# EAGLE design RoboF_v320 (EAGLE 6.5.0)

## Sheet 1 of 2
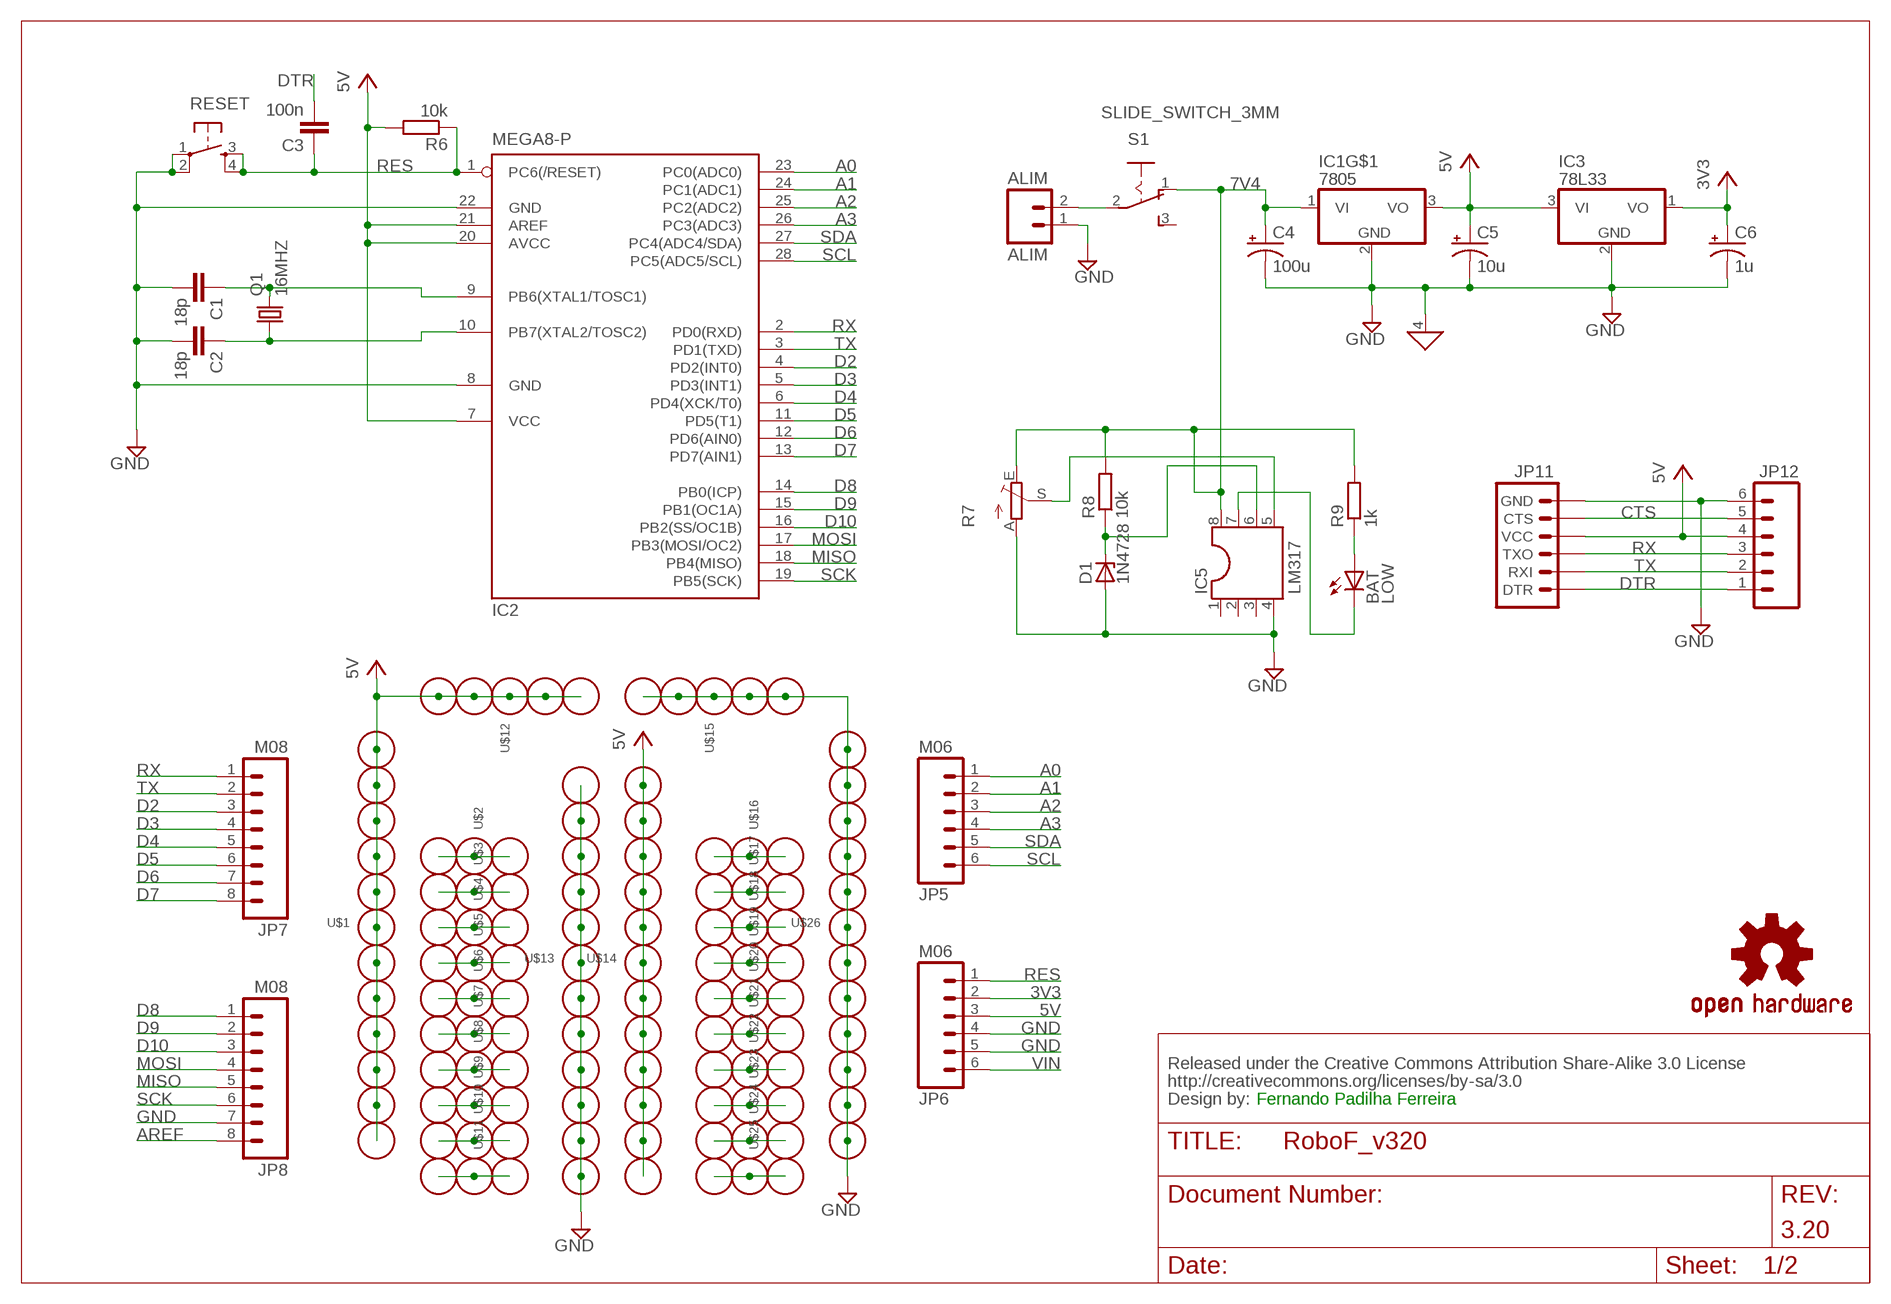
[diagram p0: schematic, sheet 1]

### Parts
ALIM  ALIM  M02POLAR  [MOLEX-1X2]
BAT  LOW  TLLG4400  [LED3MM]
C1  18p  C-EU050-024X044  [C050-024X044]
C2  18p  C-EU050-024X044  [C050-024X044]
C3  100n  C-EU050-024X044  [C050-024X044]
C4  100u  CPOL-USE2.5-6  [E2,5-6]
C5  10u  CPOL-USE2.5-6  [E2,5-6]
C6  1u  CPOL-USE2.5-5  [E2,5-5]
CC_TEXT1  CREATIVE_COMMONS  [CREATIVE_COMMONS]
D1  1N4728  [DO41Z10]
IC1  7805  [TO220H]
IC2  MEGA8-P  [DIL28-3]
IC3  78L33  78L24Z  [TO92]
IC5  LM317  DIL8  [DIL08]
JP5  M06  [1X06_FEMALE_NO_SILK]
JP6  M06  [1X06_FEMALE_NO_SILK]
JP7  M08  [1X08_FEMALE_NO_SILK]
JP8  M08  [1X08_FEMALE_NO_SILK]
JP11  ARDUINO_SERIAL_PROGRAMPTH  [1X06]
JP12  M06SIP  [1X06]
LOGO1  OSHW-LOGOL  [OSHW-LOGO-L]
Q1  16MHZ  CRYSTALHC49S  [HC49/S]
R6  10k  R-EU_0207/7  [0207/7]
R7  TRIM_EU-RS3  [RS3]
R8  10k  R-EU_0207/7  [0207/7]
R9  1k  R-EU_0207/7  [0207/7]
RESET  TAC_SWITCHPTH  [TACTILE-PTH]
S1  SLIDE_SWITCH_3MM  [SS3MM]
U$1  WIREPAD-12X1  [12X-1,6/0,9]
U$2  WIREPAD-3X1  [3X-1,6/0,9]
U$3  WIREPAD-3X1  [3X-1,6/0,9]
U$4  WIREPAD-3X1  [3X-1,6/0,9]
U$5  WIREPAD-3X1  [3X-1,6/0,9]
U$6  WIREPAD-3X1  [3X-1,6/0,9]
U$7  WIREPAD-3X1  [3X-1,6/0,9]
U$8  WIREPAD-3X1  [3X-1,6/0,9]
U$9  WIREPAD-3X1  [3X-1,6/0,9]
U$10  WIREPAD-3X1  [3X-1,6/0,9]
U$11  WIREPAD-3X1  [3X-1,6/0,9]
U$12  WIREPAD-5X1  [5X-1,6/0,9]
U$13  WIREPAD-12X1  [12X-1,6/0,9]
U$14  WIREPAD-12X1  [12X-1,6/0,9]
U$15  WIREPAD-5X1  [5X-1,6/0,9]
U$16  WIREPAD-3X1  [3X-1,6/0,9]
U$17  WIREPAD-3X1  [3X-1,6/0,9]
U$18  WIREPAD-3X1  [3X-1,6/0,9]
U$19  WIREPAD-3X1  [3X-1,6/0,9]
U$20  WIREPAD-3X1  [3X-1,6/0,9]
U$21  WIREPAD-3X1  [3X-1,6/0,9]
U$22  WIREPAD-3X1  [3X-1,6/0,9]
U$23  WIREPAD-3X1  [3X-1,6/0,9]
U$24  WIREPAD-3X1  [3X-1,6/0,9]
U$25  WIREPAD-3X1  [3X-1,6/0,9]
U$26  WIREPAD-12X1  [12X-1,6/0,9]

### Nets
3V3: C6.+ IC3.1(VO) JP6.2 ; also sheet 2
5V: C5.+ IC1.3(VO) IC2.7(VCC) IC2.20(AVCC) IC2.21(AREF) IC3.3(VI) JP6.3 JP11.4(VCC) JP12.4 R6.2 U$1.P$1 U$1.P$2 U$1.P$3 U$1.P$4 U$1.P$5 U$1.P$6 U$1.P$7 U$1.P$8 U$1.P$9 U$1.P$10 U$1.P$11 U$1.P$12 U$12.P$1(P$) U$12.P$2 U$12.P$3 U$12.P$4 U$12.P$5 U$14.P$1 U$14.P$2 U$14.P$3 U$14.P$4 U$14.P$5 U$14.P$6 U$14.P$7 U$14.P$8 U$14.P$9 U$14.P$10 U$14.P$11 U$14.P$12 ; also sheet 2
7V4 [MTR]: C4.+ IC1.1(VI) IC5.8 R7.E R8.2 R9.2 S1.1(O) ; also sheet 2
A0 [SIGNAL]: IC2.23(PC0(ADC0)) JP5.1 ; also sheet 2
A1 [SIGNAL]: IC2.24(PC1(ADC1)) JP5.2 ; also sheet 2
A2 [SIGNAL]: IC2.25(PC2(ADC2)) JP5.3 ; also sheet 2
A3 [SIGNAL]: IC2.26(PC3(ADC3)) JP5.4 ; also sheet 2
AREF: JP8.8
CTS [SIGNAL]: JP11.5(CTS) JP12.5
D2 [SIGNAL]: IC2.4(PD2(INT0)) JP7.3 ; also sheet 2
D3 [SIGNAL]: IC2.5(PD3(INT1)) JP7.4 ; also sheet 2
D4 [SIGNAL]: IC2.6(PD4(XCK/T0)) JP7.5 ; also sheet 2
D5 [SIGNAL]: IC2.11(PD5(T1)) JP7.6 ; also sheet 2
D6 [SIGNAL]: IC2.12(PD6(AIN0)) JP7.7 ; also sheet 2
D7 [SIGNAL]: IC2.13(PD7(AIN1)) JP7.8 ; also sheet 2
D8 [SIGNAL]: IC2.14(PB0(ICP)) JP8.1 ; also sheet 2
D9 [SIGNAL]: IC2.15(PB1(OC1A)) JP8.2 ; also sheet 2
D10 [SIGNAL]: IC2.16(PB2(SS/OC1B)) JP8.3 ; also sheet 2
DTR [SIGNAL]: C3.2 JP11.1(DTR) JP12.1
GND: ALIM.1 C1.2 C2.2 C4.- C5.- C6.- D1.A IC1.2(GND) IC1.4(GND) IC2.8(GND) IC2.22(GND) IC3.2(GND) IC5.4 JP6.4 JP6.5 JP8.7 JP11.6(GND) JP12.6 R7.A RESET.1 RESET.2 U$13.P$1 U$13.P$2 U$13.P$3 U$13.P$4 U$13.P$5 U$13.P$6 U$13.P$7 U$13.P$8 U$13.P$9 U$13.P$10 U$13.P$11 U$13.P$12 U$15.P$1(P$) U$15.P$2 U$15.P$3 U$15.P$4 U$15.P$5 U$26.P$1 U$26.P$2 U$26.P$3 U$26.P$4 U$26.P$5 U$26.P$6 U$26.P$7 U$26.P$8 U$26.P$9 U$26.P$10 U$26.P$11 U$26.P$12 ; also sheet 2
GND1: BAT.K(C) IC5.7
MISO [SIGNAL]: IC2.18(PB4(MISO)) JP8.5 ; also sheet 2
MOSI [SIGNAL]: IC2.17(PB3(MOSI/OC2)) JP8.4 ; also sheet 2
N$6 [SIGNAL]: C2.1 IC2.10(PB7(XTAL2/TOSC2)) Q1.1
N$8 [MTR]: ALIM.2 S1.2(P)
N$11 [SIGNAL]: C1.1 IC2.9(PB6(XTAL1/TOSC1)) Q1.2
N$55: U$3.P$1 U$3.P$2 U$3.P$3
N$56: U$4.P$1 U$4.P$2 U$4.P$3
N$57: U$5.P$1 U$5.P$2 U$5.P$3
N$58: U$6.P$1 U$6.P$2 U$6.P$3
N$59: U$7.P$1 U$7.P$2 U$7.P$3
N$70: U$8.P$1 U$8.P$2 U$8.P$3
N$80: U$9.P$1 U$9.P$2 U$9.P$3
N$88: U$10.P$1 U$10.P$2 U$10.P$3
N$89: U$11.P$1 U$11.P$2 U$11.P$3
N$92: U$17.P$1 U$17.P$2 U$17.P$3
N$93: U$18.P$1 U$18.P$2 U$18.P$3
N$94: U$19.P$1 U$19.P$2 U$19.P$3
N$115: U$20.P$1 U$20.P$2 U$20.P$3
N$116: U$21.P$1 U$21.P$2 U$21.P$3
N$117: U$22.P$1 U$22.P$2 U$22.P$3
N$120: U$23.P$1 U$23.P$2 U$23.P$3
N$121: U$24.P$1 U$24.P$2 U$24.P$3
N$122: U$25.P$1 U$25.P$2 U$25.P$3
N$124: U$2.P$1 U$2.P$2 U$2.P$3
N$126: U$16.P$1 U$16.P$2 U$16.P$3
N$185 [SIGNAL]: BAT.A R9.1
N$189: D1.C IC5.6 R8.1
N$190: IC5.5 R7.S
RES [SIGNAL]: C3.1 IC2.1(PC6(/RESET)) JP6.1 R6.1 RESET.3 RESET.4 ; also sheet 2
RX [SIGNAL]: IC2.2(PD0(RXD)) JP7.1 JP11.3(TXO) JP12.3 ; also sheet 2
SCK [SIGNAL]: IC2.19(PB5(SCK)) JP8.6 ; also sheet 2
SCL [SIGNAL]: IC2.28(PC5(ADC5/SCL)) JP5.6 ; also sheet 2
SDA [SIGNAL]: IC2.27(PC4(ADC4/SDA)) JP5.5 ; also sheet 2
TX [SIGNAL]: IC2.3(PD1(TXD)) JP7.2 JP11.2(RXI) JP12.2 ; also sheet 2
VIN: JP6.6
Unconnected: IC5.1 IC5.2 IC5.3 S1.3(S)

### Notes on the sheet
- Fernando Padilha Ferreira
- 3.20

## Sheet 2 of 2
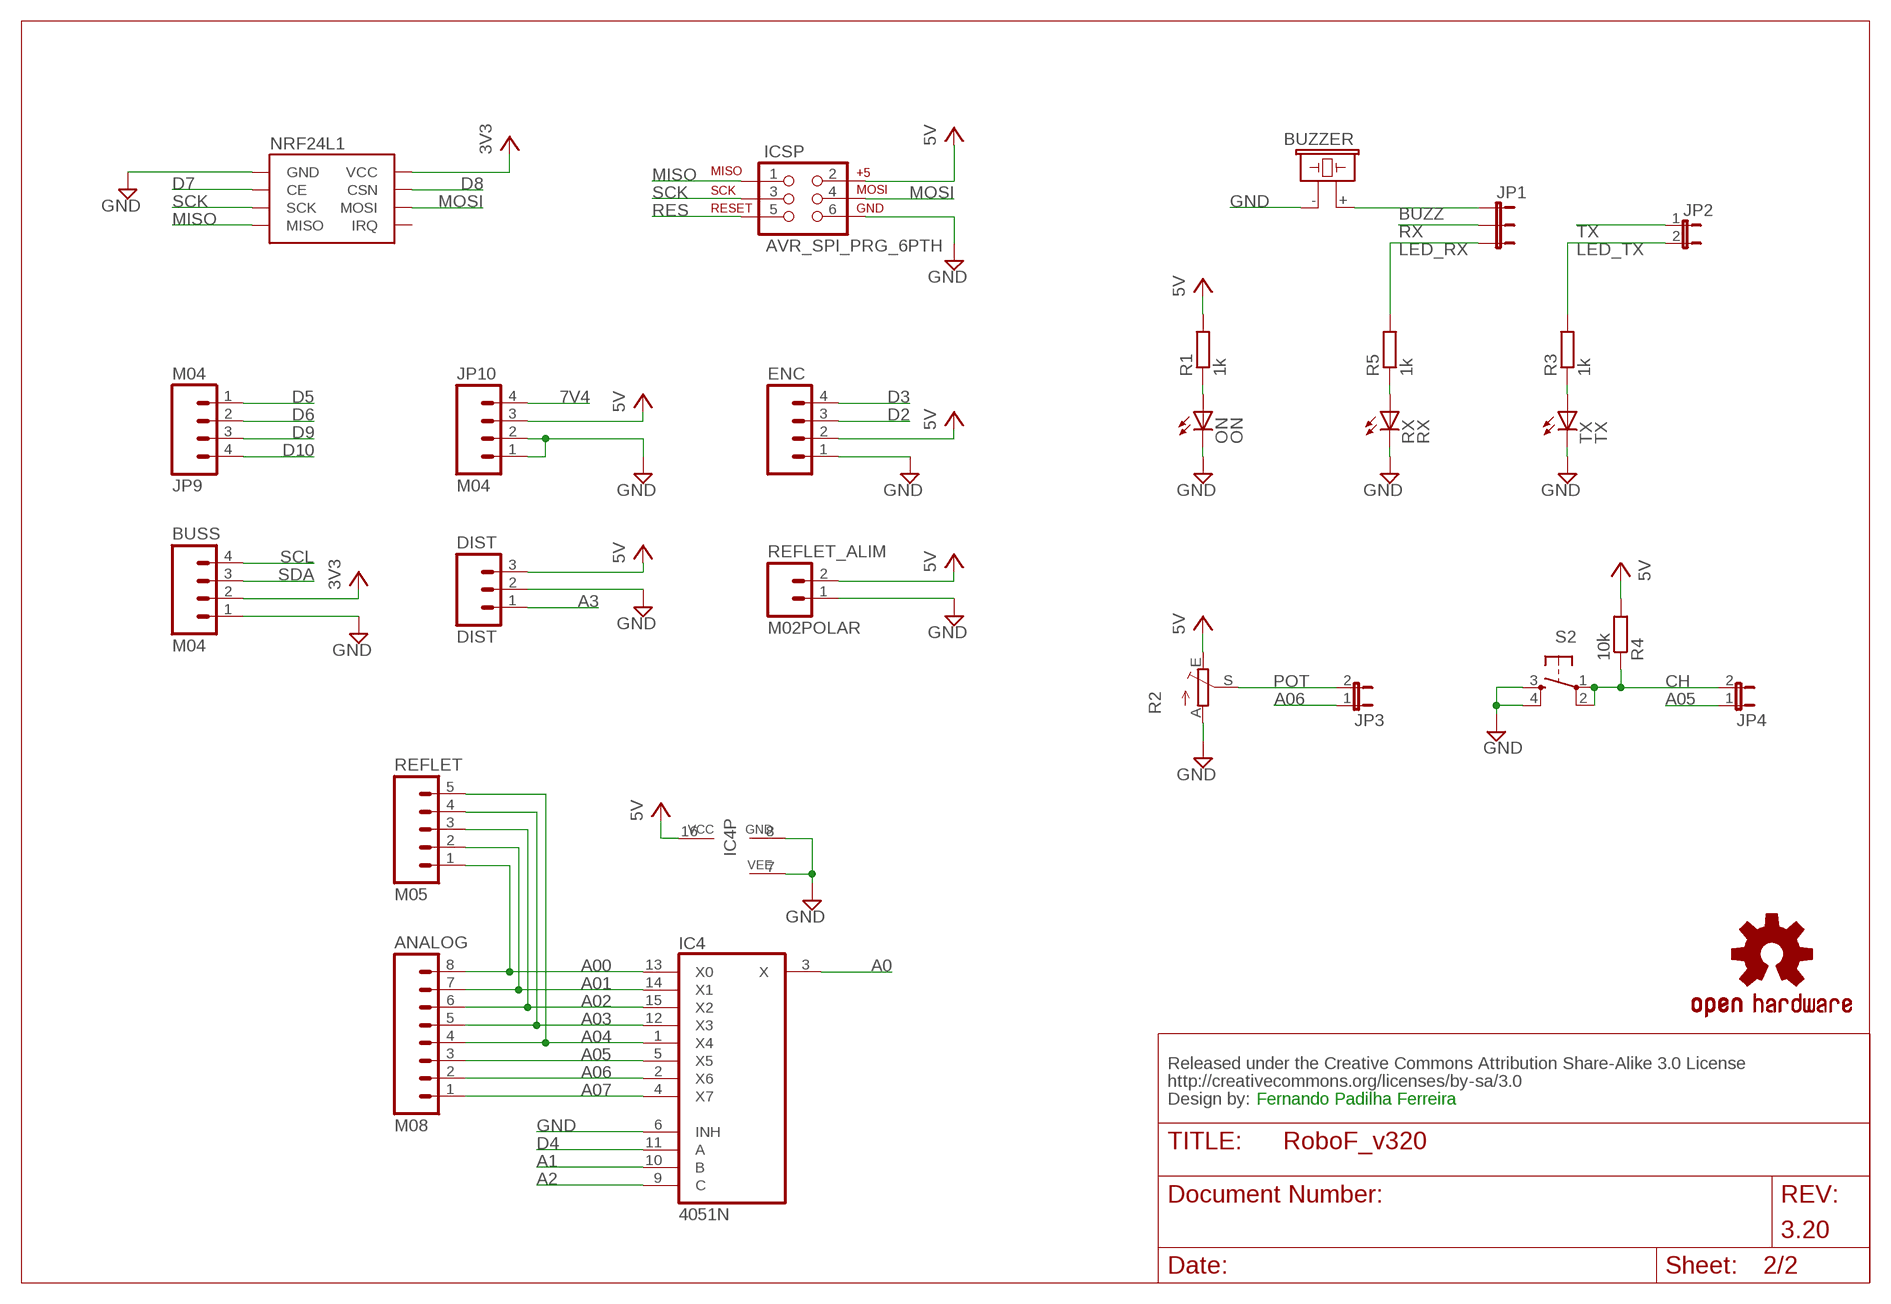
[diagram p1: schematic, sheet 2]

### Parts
ANALOG  M08  [1X08_FEMALE_NO_SILK]
BUSS  M04  [1X04_FEMALE]
BUZZER  F/CM12P  [F/CM12P]
CC_TEXT2  CREATIVE_COMMONS  [CREATIVE_COMMONS]
DIST  DIST  M03POLAR  [MOLEX-1X3]
ENC  M04POLAR  [MOLEX-1X4]
IC4  4051N  [DIL16]
ICSP  AVR_SPI_PRG_6PTH  [2X3]
JP1  JUMPER-3PTH  [1X03]
JP2  JUMPER-2PTH  [1X02]
JP3  JUMPER-2PTH  [1X02]
JP4  JUMPER-2PTH  [1X02]
JP9  M04  [1X04_FEMALE]
JP10  M04  [1X04_FEMALE]
LOGO2  OSHW-LOGOL  [OSHW-LOGO-L]
NRF24L1  NRF24L01  [NRF24L01]
ON  ON  TLLG4400  [LED3MM]
R1  1k  R-EU_0207/7  [0207/7]
R2  TRIM_EU-RS3  [RS3]
R3  1k  R-EU_0207/7  [0207/7]
R4  10k  R-EU_0207/7  [0207/7]
R5  1k  R-EU_0207/7  [0207/7]
REFLET  M05  [MOLEX-1X5]
REFLET_ALIM  M02POLAR  [MOLEX-1X2]
RX  RX  TLLR4400  [LED3MM]
S2  TAC_SWITCHPTH  [TACTILE-PTH]
TX  TX  TLLR4400  [LED3MM]

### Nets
3V3: BUSS.2 NRF24L1.2(VCC) ; also sheet 1
5V: DIST.3 ENC.2 IC4.16(VCC) ICSP.2 JP10.3 R1.2 R2.E R4.2 REFLET_ALIM.2 ; also sheet 1
7V4 [MTR]: JP10.4 ; also sheet 1
A0 [SIGNAL]: IC4.3(X) ; also sheet 1
A00 [SIGNAL]: ANALOG.8 IC4.13(X0) REFLET.1
A1 [SIGNAL]: IC4.10(B) ; also sheet 1
A01 [SIGNAL]: ANALOG.7 IC4.14(X1) REFLET.2
A2 [SIGNAL]: IC4.9(C) ; also sheet 1
A02 [SIGNAL]: ANALOG.6 IC4.15(X2) REFLET.3
A3 [SIGNAL]: DIST.1 ; also sheet 1
A03 [SIGNAL]: ANALOG.5 IC4.12(X3) REFLET.4
A04 [SIGNAL]: ANALOG.4 IC4.1(X4) REFLET.5
A05 [SIGNAL]: ANALOG.3 IC4.5(X5) JP4.1
A06 [SIGNAL]: ANALOG.2 IC4.2(X6) JP3.1
A07 [SIGNAL]: ANALOG.1 IC4.4(X7)
BUZZ [SIGNAL]: BUZZER.+ JP1.1
CH [SIGNAL]: JP4.2 R4.1 S2.1 S2.2
D2 [SIGNAL]: ENC.3 ; also sheet 1
D3 [SIGNAL]: ENC.4 ; also sheet 1
D4 [SIGNAL]: IC4.11(A) ; also sheet 1
D5 [SIGNAL]: JP9.1 ; also sheet 1
D6 [SIGNAL]: JP9.2 ; also sheet 1
D7 [SIGNAL]: NRF24L1.3(CE) ; also sheet 1
D8 [SIGNAL]: NRF24L1.4(CSN) ; also sheet 1
D9 [SIGNAL]: JP9.3 ; also sheet 1
D10 [SIGNAL]: JP9.4 ; also sheet 1
GND: BUSS.1 BUZZER.- DIST.2 ENC.1 IC4.6(INH) IC4.7(VEE) IC4.8(GND) ICSP.6 JP10.1 JP10.2 NRF24L1.1(GND) ON.K(C) R2.A REFLET_ALIM.1 RX.K(C) S2.3 S2.4 TX.K(C) ; also sheet 1
LED_RX [SIGNAL]: JP1.3 R5.2
LED_TX [SIGNAL]: JP2.2 R3.2
MISO [SIGNAL]: ICSP.1 NRF24L1.7(MISO) ; also sheet 1
MOSI [SIGNAL]: ICSP.4 NRF24L1.6(MOSI) ; also sheet 1
N$1 [SIGNAL]: R3.1 TX.A
N$2 [SIGNAL]: R5.1 RX.A
N$186 [SIGNAL]: ON.A R1.1
POT [SIGNAL]: JP3.2 R2.S
RES [SIGNAL]: ICSP.5 ; also sheet 1
RX [SIGNAL]: JP1.2 ; also sheet 1
SCK [SIGNAL]: ICSP.3 NRF24L1.5(SCK) ; also sheet 1
SCL [SIGNAL]: BUSS.4 ; also sheet 1
SDA [SIGNAL]: BUSS.3 ; also sheet 1
TX [SIGNAL]: JP2.1 ; also sheet 1
Unconnected: NRF24L1.8(IRQ)

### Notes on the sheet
- Fernando Padilha Ferreira
- 3.20

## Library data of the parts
ALIM = SparkFun:M02: Header 2
ANALOG JP7 JP8 = FernandoLib:M08
BAT ON = led:TLLG4400: Low Current (2mA) LED 3 mm Tinted Diffused Package color GREEN; MF: VISHAY SEMICONDUCTOR; OC_FARNELL: 1612435
BUSS JP9 JP10 = FernandoLib:M04
BUZZER = buzzer:F/CM12P: BUZZER; OC_FARNELL: unknown; OC_NEWARK: unknown
C1-C3 = rcl:C-EU: CAPACITOR, European symbol
C4 C5 = rcl:CPOL-US: POLARIZED CAPACITOR, American symbol
C6 = resistor:CPOL-US: POLARIZED CAPACITOR, American symbol
CC_TEXT1 CC_TEXT2 = SparkFun-Aesthetics:CREATIVE_COMMONS: Creative Commons License summary
D1 = diode:1N4728: Z DIODE
DIST = SparkFun-Connectors:M03: Header 3 Standard 3-pin 0.1" header. Use with straight break away headers (SKU : PRT-00116), right angle break away headers (PRT-00553), swiss pins (PRT-00743), machine pins (PRT-00117), and female headers (PRT-00115). Molex polarized connector foot print use with SKU : PRT-08232 with associated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
ENC = SparkFun-Connectors:M04: Header 4 Standard 4-pin 0.1" header. Use with straight break away headers (SKU : PRT-00116), right angle break away headers (PRT-00553), swiss pins (PRT-00743), machine pins (PRT-00117), and female headers (PRT-00115). Molex polarized connector foot print use with SKU : PRT-08231 with associated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
IC1 = FernandoLib:78*
IC2 = atmel:MEGA8-P: MICROCONTROLLER 8 Kbytes FLASH, 1 kbytes SRAM, 512 bytes EEPROM, USART, 4-channel 10 bit ADC, 2-channel 8 bit ADC Pin compatible with Atmega48, ATMega88, ATMega168 Source: avr.lbr; OC_FARNELL: unknown; OC_NEWARK: unknown
IC3 = linear:78*: Positive VOLTAGE REGULATOR Source: http://cache.national.com/ds/LM/LM78L05.pdf http://www.fairchildsemi.com/ds/LM/LM7805.pdf
IC4 = 40xx:4051: 8-channel ANALOG MULTIPLEXER
IC5 = ic-package:DIL8: Dual In Line / Socket
ICSP = SparkFun-Connectors:AVR_SPI_PRG_6: AVR ISP 6 Pin This is the reduced ISP connector for AVR programming. Common on Arduino. This footprint will take up less PCB space and can be used with a 10-pin to 6-pin adapter such as SKU: BOB-08508
JP1 = SparkFun-Passives:JUMPER-3
JP2-JP4 = SparkFun-Passives:JUMPER-2: Jumper
JP5 JP6 = FernandoLib:M06
JP11 = SparkFun-Connectors:ARDUINO_SERIAL_PROGRAM: FTDI connector footprints
JP12 = SparkFun-Connectors:M06: Header 6 Standard 6-pin 0.1" header. Use with straight break away headers (SKU : PRT-00116), right angle break away headers (PRT-00553), swiss pins (PRT-00743), machine pins (PRT-00117), and female headers (PRT-00115). Molex polarized connector foot print use with SKU : PRT-08094 with associated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
LOGO1 LOGO2 = SparkFun-Aesthetics:OSHW-LOGO: Open Source Hardware Logo This logo indicates the piece of hardware it is found on incorporates a OSHW license and/or adheres to the definition of open source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
NRF24L1 = FernandoLib:NRF24L01
Q1 = crystal:CRYSTAL: CRYSTAL; OC_FARNELL: 1667008; OC_NEWARK: unknown
R1 R3-R6 R8 R9 = resistor:R-EU_: RESISTOR, European symbol
R2 R7 = pot:TRIM_EU-: POTENTIOMETER
REFLET = FernandoLib:M05
REFLET_ALIM = SparkFun-Connectors:M02: Standard 2-pin 0.1" header. Use with
RESET S2 = SparkFun:TAC_SWITCH: Momentary Switch Button commonly used for reset or general input. Spark Fun Electronics SKU : COM-00097
RX TX = led:TLLR4400: Low Current (2mA) LED 3 mm Tinted Diffused Package color RED; MF: VISHAY SEMICONDUCTOR; OC_FARNELL: 1612437
S1 = FernandoLib:SLIDE_SWITCH_3MM
U$1 U$13 U$14 U$26 = FernandoLib:WIREPAD-12X1
U$2-U$11 U$16-U$25 = FernandoLib:WIREPAD-3X1
U$12 U$15 = FernandoLib:WIREPAD-5X1

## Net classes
0 GND: width 0.762 mm, clearance 0.406 mm
1 MTR: width 1.016 mm, clearance 0.406 mm

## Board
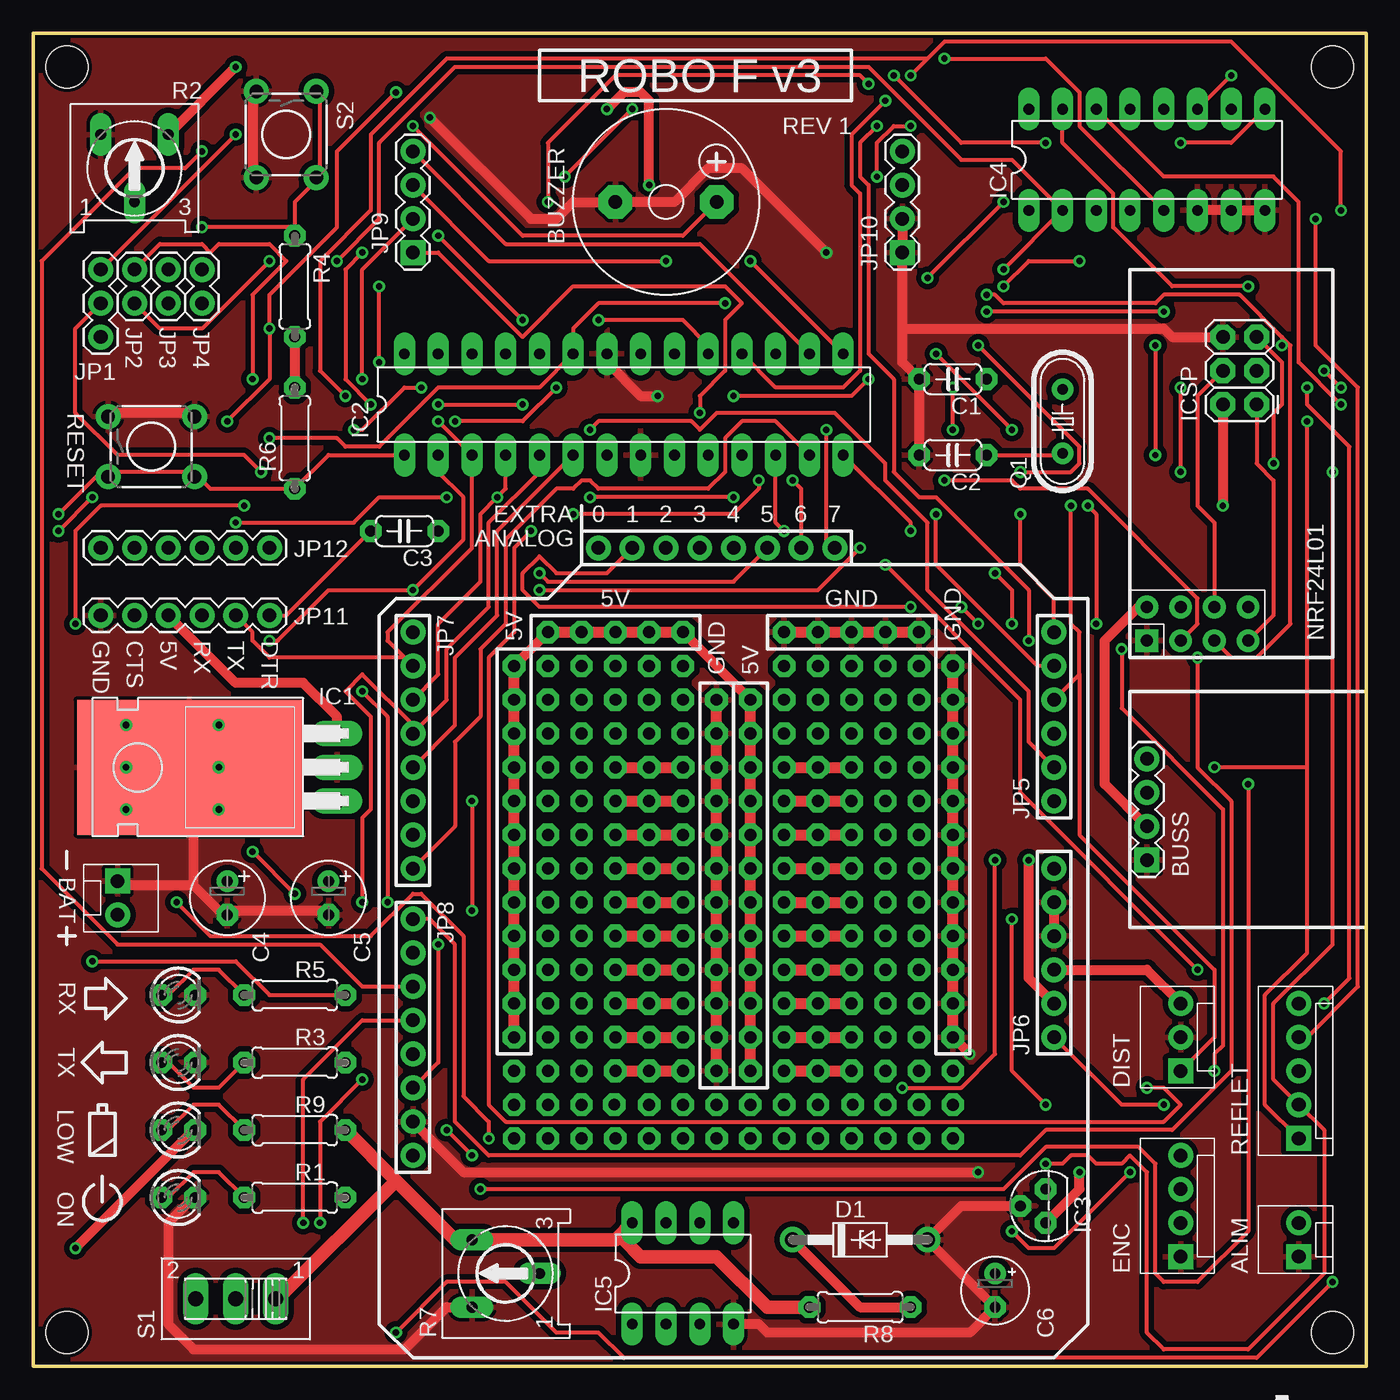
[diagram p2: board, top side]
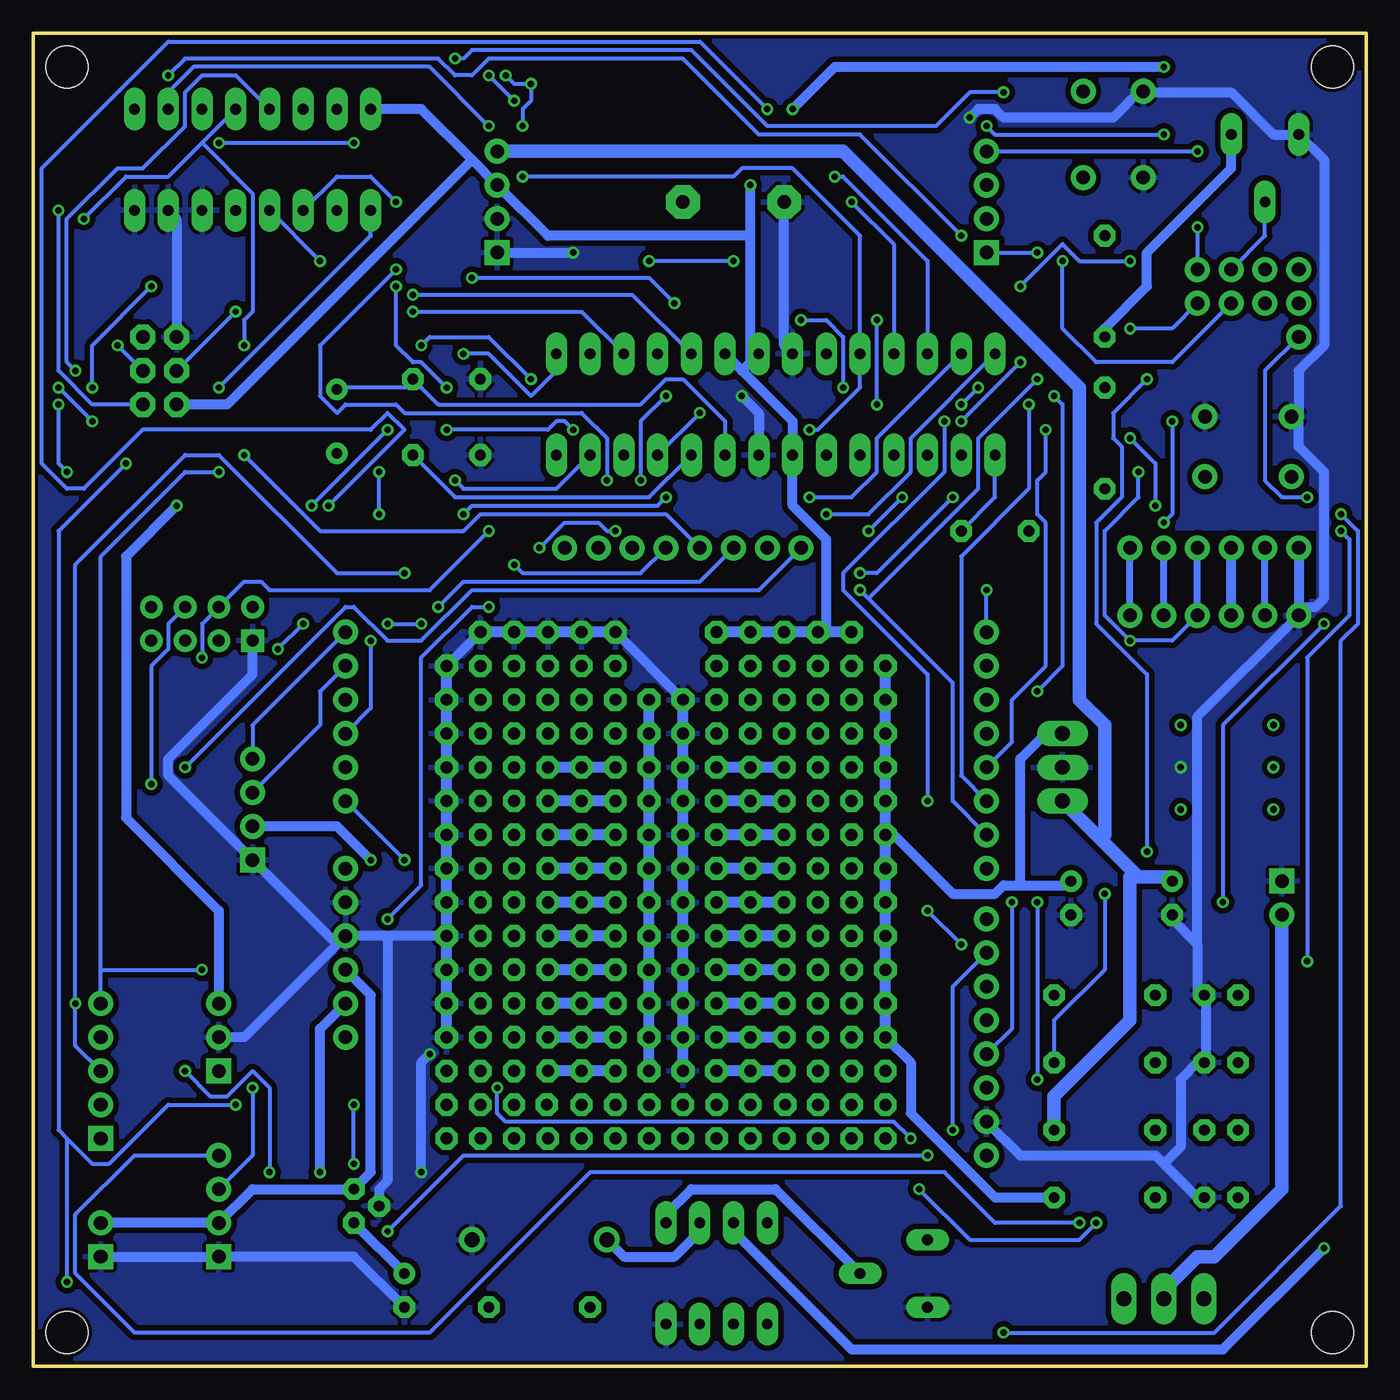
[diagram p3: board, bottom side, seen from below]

Size 100.33 x 100.33 mm. Coordinates in mm from the lower left corner, seen from the top.
Outline: 0,0 100.33,0 100.33,100.33 0,100.33 0,0
Copper layers (1*16): Top 0.035mm / dielectric 1.5mm / Bottom 0.035mm
Design rules "peteco": minimum track width 12mil, minimum drill 19mil, track to track 10mil, track to pad 10mil, pad to pad 10mil, via to via 10mil, smd to smd 0mil, copper to edge 10mil, drill to drill 8mil, minimum pad ring 16mil, minimum via ring 8mil, stop-mask expansion 4mil, vias tented up to drill 0mil, thermal gap 10mil
Holes 3.2 mm at 97.79,2.54 97.79,97.79 2.54,2.54 2.54,97.79
tRestrict: area 3.8,57.8 to 19.1,62.9
bRestrict: area 3.8,57.8 to 19.1,62.9
vRestrict: area 38.1,95.2 to 61.6,99.1

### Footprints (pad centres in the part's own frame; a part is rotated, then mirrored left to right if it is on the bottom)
MOLEX-1X2 = drill 1.016 pad 1.88 square: 1 0,0 | drill 1.016 pad 1.88: 2 2.54,0
1X08_FEMALE_NO_SILK = drill 1.016 pad 1.88: 1 0,0; 2 2.54,0; 3 5.08,0; 4 7.62,0; 5 10.16,0; 6 12.7,0; 7 15.24,0; 8 17.78,0
LED3MM = drill 0.813 octagon: A -1.27,0; K 1.27,0
1X04_FEMALE = drill 1.016 pad 1.88 square: 1 0,0 | drill 1.016 pad 1.88: 2 2.54,0; 3 5.08,0; 4 7.62,0
F/CM12P = drill 1.016 pad 2.54 octagon: + 3.81,0; - -3.81,0
C050-024X044 = drill 0.813 octagon: 1 -2.54,0; 2 2.54,0
E2,5-6 = drill 0.813 pad 1.6: + -1.27,0 | drill 0.813 pad 1.6 octagon: - 1.27,0
E2,5-5 = drill 0.813 pad 1.6: + -1.27,0 | drill 0.813 pad 1.6 octagon: - 1.27,0
DO41Z10 = drill 1.118: A 5.08,0; C -5.08,0
MOLEX-1X3 = drill 1.016 pad 1.88 square: 1 0,0 | drill 1.016 pad 1.88: 2 2.54,0; 3 5.08,0
MOLEX-1X4 = drill 1.016 pad 1.88 square: 1 0,0 | drill 1.016 pad 1.88: 2 2.54,0; 3 5.08,0; 4 7.62,0
TO220H = drill 1.118 long: 1 -2.54,-10.16; 2 0,-10.16; 3 2.54,-10.16 | smd 10.16 x 16.875: 4 0,0.953
DIL28-3 = drill 0.813 long: 1 -16.51,-3.81; 2 -13.97,-3.81; 3 -11.43,-3.81; 4 -8.89,-3.81; 5 -6.35,-3.81; 6 -3.81,-3.81; 7 -1.27,-3.81; 8 1.27,-3.81; 9 3.81,-3.81; 10 6.35,-3.81; 11 8.89,-3.81; 12 11.43,-3.81; 13 13.97,-3.81; 14 16.51,-3.81; 15 16.51,3.81; 16 13.97,3.81; 17 11.43,3.81; 18 8.89,3.81; 19 6.35,3.81; 20 3.81,3.81; 21 1.27,3.81; 22 -1.27,3.81; 23 -3.81,3.81; 24 -6.35,3.81; 25 -8.89,3.81; 26 -11.43,3.81; 27 -13.97,3.81; 28 -16.51,3.81
TO92 = drill 0.813 octagon: 1 -1.27,0; 2 0,1.905; 3 1.27,0
DIL16 = drill 0.813 long: 1 -8.89,-3.81; 2 -6.35,-3.81; 3 -3.81,-3.81; 4 -1.27,-3.81; 5 1.27,-3.81; 6 3.81,-3.81; 7 6.35,-3.81; 8 8.89,-3.81; 9 8.89,3.81; 10 6.35,3.81; 11 3.81,3.81; 12 1.27,3.81; 13 -1.27,3.81; 14 -3.81,3.81; 15 -6.35,3.81; 16 -8.89,3.81
DIL08 = drill 0.813 long: 1 -3.81,-3.81; 2 -1.27,-3.81; 3 1.27,-3.81; 4 3.81,-3.81; 5 3.81,3.81; 6 1.27,3.81; 7 -1.27,3.81; 8 -3.81,3.81
2X3 = drill 1.016 pad 1.88 octagon: 1 0,0; 2 0,2.54; 3 2.54,0; 4 2.54,2.54; 5 5.08,0; 6 5.08,2.54
1X03 = drill 1.016 pad 1.88: 1 0,0; 2 2.54,0; 3 5.08,0
1X02 = drill 1.016 pad 1.88: 1 0,0; 2 2.54,0
1X06_FEMALE_NO_SILK = drill 1.016 pad 1.88: 1 0,0; 2 2.54,0; 3 5.08,0; 4 7.62,0; 5 10.16,0; 6 12.7,0
1X06 = drill 1.016 pad 1.88: 1 0,0; 2 2.54,0; 3 5.08,0; 4 7.62,0; 5 10.16,0; 6 12.7,0
NRF24L01 = drill 0.9 pad 1.676 square: 1 0,0 | drill 0.9 pad 1.676: 2 -2.54,0; 3 0,2.54; 4 -2.54,2.54; 5 0,5.08; 6 -2.54,5.08; 7 0,7.62; 8 -2.54,7.62
HC49/S = drill 0.813: 1 -2.413,0; 2 2.413,0
0207/7 = drill 0.813 octagon: 1 -3.81,0; 2 3.81,0
RS3 = drill 0.813 long: A -2.54,2.54; E 2.54,2.54; S 0,-2.54
MOLEX-1X5 = drill 1.016 pad 1.88 square: 1 0,0 | drill 1.016 pad 1.88: 2 2.54,0; 3 5.08,0; 4 7.62,0; 5 10.16,0
TACTILE-PTH = drill 1.016 pad 1.88: 1 -3.251,2.261; 2 3.251,2.261; 3 -3.251,-2.261; 4 3.251,-2.261
SS3MM = drill 1.118 long: 1 -3,0; 2 0,0; 3 3,0
12X-1,6/0,9 = drill 0.9 pad 1.676 octagon: P$1 -12.7,0; P$2 -10.16,0; P$3 -7.62,0; P$4 -5.08,0; P$5 -2.54,0; P$6 0,0; P$7 2.54,0; P$8 5.08,0; P$9 7.62,0; P$10 10.16,0; P$11 12.7,0; P$12 15.24,0
3X-1,6/0,9 = drill 0.9 pad 1.676 octagon: P$1 -2.54,0; P$2 0,0; P$3 2.54,0
5X-1,6/0,9 = drill 0.9 pad 1.676 octagon: P$1 -5.08,0; P$2 -2.54,0; P$3 0,0; P$4 2.54,0; P$5 5.08,0

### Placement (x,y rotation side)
ALIM  6.35,36.51 270 top
ANALOG  60.33,61.59 180 top
BAT  10.92,17.78 0 top
BUSS  83.82,38.1 90 top
BUZZER  47.62,87.63 0 top
C1  69.22,74.3 180 top
C2  69.22,68.58 180 top
C3  27.94,62.87 180 top
C4  14.61,35.24 270 top
C5  22.23,35.24 270 top
C6  72.39,5.71 270 top
CC_TEXT1  not placed on the board
CC_TEXT2  not placed on the board
D1  62.23,9.53 0 top
DIST  86.36,22.23 90 top
ENC  86.36,8.26 90 top
IC1  12.7,45.09 90 top
IC2  44.45,72.39 0 top
IC3  76.2,12.06 90 top
IC4  83.82,90.81 0 top
IC5  48.9,6.99 0 top
ICSP  92.08,72.39 90 top
JP1  5.08,82.55 270 top
JP2  7.62,80.01 90 top
JP3  10.16,80.01 90 top
JP4  12.7,80.01 90 top
JP5  76.83,42.55 90 top
JP6  76.83,24.77 90 top
JP7  28.57,55.24 270 top
JP8  28.57,33.66 270 top
JP9  28.57,83.82 90 top
JP10  65.41,83.82 90 top
JP11  17.78,56.52 180 top
JP12  17.78,61.59 180 top
LOGO1  not placed on the board
LOGO2  not placed on the board
NRF24L1  83.82,54.61 270 top
ON  10.92,12.7 0 top
Q1  77.47,71.12 90 top
R1  19.68,12.7 0 top
R2  7.62,90.17 0 top
R3  19.68,22.86 0 top
R4  19.68,81.28 270 top
R5  19.68,27.94 0 top
R6  19.68,69.85 90 top
R7  35.56,6.99 90 top
R8  62.23,4.45 180 top
R9  19.68,17.78 0 top
REFLET  95.25,17.14 90 top
REFLET_ALIM  95.25,8.26 90 top
RESET  8.89,69.22 0 top
RX  10.92,27.94 0 top
S1  15.24,5.08 180 top
S2  19.05,92.71 270 top
TX  10.92,22.86 0 top
U$1  36.2,37.47 90 top
U$2  59.05,24.77 0 top
U$3  46.35,45.09 0 top
U$4  46.35,42.55 0 top
U$5  46.35,40.01 0 top
U$6  46.35,37.47 0 top
U$7  46.35,34.92 0 top
U$8  46.35,32.38 0 top
U$9  46.35,29.84 0 top
U$10  46.35,27.3 0 top
U$11  46.35,24.77 0 top
U$12  43.81,55.24 0 top
U$13  51.44,34.92 90 top
U$14  53.98,34.92 90 top
U$15  61.59,55.24 0 top
U$16  59.05,22.23 0 top
U$17  46.35,22.23 0 top
U$18  59.05,45.09 0 top
U$19  59.05,42.55 0 top
U$20  59.05,40.01 0 top
U$21  59.05,37.47 0 top
U$22  59.05,34.92 0 top
U$23  59.05,32.38 0 top
U$24  59.05,29.84 0 top
U$25  59.05,27.3 0 top
U$26  69.22,37.47 90 top

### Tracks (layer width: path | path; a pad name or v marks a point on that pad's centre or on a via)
3V3  (via drill 0.48)
  Top 0.762: NRF24L1.2 83.19,57.15 80.64,54.61 80.64,43.81 BUSS.2 | v78.74,14.61 78.74,13.34 IC3.1 | v74.93,38.1 74.93,29.21 JP6.2
  Bottom 0.762: IC3.1 C6.+ | JP6.2 78.74,25.4 v78.74,14.61 | BUSS.2 77.47,40.64 v74.93,38.1
5V  (via drill 0.48)
  Top 0.762: DIST.3 83.82,29.84 JP6.3 | ICSP.2 v89.53,64.77 | JP11.4 15.24,51.44 20.32,51.44 22.86,48.9 IC1.3 | R4.2 R6.2 | U$14.P$3 U$14.P$1 | U$14.P$4 U$14.P$1 | U$14.P$5 U$14.P$1 | U$14.P$6 U$14.P$1 | U$14.P$7 U$14.P$1 | U$14.P$8 U$14.P$1 | U$14.P$9 U$14.P$1 | U$14.P$10 U$14.P$1 | U$14.P$11 U$14.P$1 | U$12.P$2 U$12.P$1 | U$12.P$3 U$12.P$1 | U$12.P$4 U$12.P$1 | U$1.P$3 U$1.P$1 | U$1.P$4 U$1.P$1 | U$1.P$5 U$1.P$1 | U$1.P$6 U$1.P$1 | U$1.P$8 U$1.P$7 | U$1.P$9 U$1.P$7 | U$1.P$10 U$1.P$7 | U$1.P$11 U$1.P$7 | U$1.P$12 U$12.P$1 | U$12.P$5 U$14.P$12 | v15.24,97.79 R2.E | v43.18,94.61 44.45,95.89 45.72,95.89 46.35,95.25 v46.35,88.9 | U$1.P$7 U$1.P$1
  Bottom 0.762: JP11.4 JP12.4 | REFLET_ALIM.2 ENC.2 83.82,13.34 IC3.3 74.93,14.61 74.93,27.94 JP6.3 | IC4.16 71.12,94.61 67.31,90.81 | 67.31,90.81 JP10.3 61.59,85.09 46.35,85.09 | ICSP.2 85.72,72.39 67.31,90.81 | DIST.3 86.36,34.29 93.34,41.27 93.34,60.96 v89.53,64.77 | 26.04,36.2 27.3,36.2 27.94,35.56 31.11,35.56 36.2,40.64 U$1.P$7 | 26.04,36.2 22.23,36.2 C5.+ | IC1.3 24.13,47.62 26.04,45.72 26.04,36.2 | R2.E 10.16,90.17 16.51,83.82 16.51,81.28 19.68,78.11 R4.2 | IC2.20 46.99,74.93 | 46.99,74.93 43.18,71.12 IC2.7 43.18,64.77 40.64,62.23 40.64,55.24 U$12.P$2 | 46.99,74.93 46.35,75.56 | R1.2 27.94,12.7 34.29,19.05 34.29,22.86 U$1.P$1 | v15.24,97.79 40.01,97.79 v43.18,94.61 | 46.35,75.56 46.35,85.09 | 46.35,85.09 v46.35,88.9 | 46.35,75.56 IC2.21
7V4
  Top 1.016: 27.3,13.97 31.75,9.53 R7.E 43.81,9.53 IC5.8 44.45,9.53 45.72,8.26 51.44,8.26 55.24,4.45 R8.2 | 27.3,13.97 R9.2 | 27.3,13.97 18.41,5.08 S1.1
  Bottom 1.016: IC1.1 20,39.69 | 20,39.69 17.46,37.15 | 17.46,37.15 17.14,36.83 14.61,36.83 C4.+ | JP10.4 39.37,91.44 21.59,73.66 21.59,50.16 19.68,48.26 19.68,40.01 20,39.69 | R9.2 23.5,20.32 17.78,26.04 17.78,36.83 17.46,37.15
A0  (via drill 0.48)
  Top 0.305: v52.07,80.01 42.55,80.01 40.64,78.11 IC2.23 38.1,73.66 30.48,73.66 26.04,69.22 23.5,69.22 22.86,69.85 v17.78,69.85 | v73.03,87.63 v67.31,81.92 | v72.39,38.1 72.39,23.5 69.85,20.95 v65.41,20.95 | v34.29,17.14 34.29,18.41 32.38,20.32 32.38,32.38 29.21,35.56 28.57,35.56 25.4,32.38 13.34,32.38 v10.79,34.92 | v3.17,55.88 3.17,62.87 5.08,64.77 v15.88,64.77
  Bottom 0.305: v52.07,80.01 53.98,81.92 v67.31,81.92 | v73.03,87.63 74.93,89.53 77.47,89.53 IC4.3 | v72.39,38.1 JP5.1 | v65.41,20.95 65.41,19.05 64.77,18.41 35.56,18.41 v34.29,17.14 | v10.79,34.92 10.79,48.26 v3.17,55.88 | v15.88,64.77 15.88,67.94 v17.78,69.85
A00  (via drill 0.48)
  Top 0.305: v98.42,73.66 v97.16,74.93 | 95.89,45.09 95.89,31.11 92.71,27.94 92.71,19.68 REFLET.1 | 95.89,45.09 v95.89,71.12 | 95.89,45.09 v88.9,45.09
  Bottom 0.305: IC4.13 85.09,97.16 87.63,97.16 88.9,95.89 88.9,93.34 92.08,90.17 93.98,90.17 97.79,86.36 97.79,75.56 v97.16,74.93 | v95.89,71.12 v98.42,73.66 | ANALOG.8 45.72,58.42 67.31,58.42 71.12,54.61 73.66,54.61 76.2,57.15 76.83,57.15 v88.9,45.09
A1  (via drill 0.48)
  Top 0.305: v41.91,70.48 42.55,71.12 49.53,71.12 50.16,70.48 51.44,71.75 60.33,71.75 64.14,67.94 64.14,66.67 67.31,63.5 67.31,58.42 74.93,50.8 74.93,46.99 JP5.2 | v66.04,93.34 64.77,93.34 63.5,92.08 v63.5,89.53
  Bottom 0.305: v41.91,70.48 41.27,70.48 38.1,73.66 IC2.24 38.1,85.09 43.18,90.17 46.99,90.17 47.62,89.53 v63.5,89.53 | IC4.10 90.17,95.89 88.27,97.79 70.48,97.79 v66.04,93.34
A01  (via drill 0.48)
  Top 0.305: IC4.14 85.09,89.53 93.34,89.53 95.25,87.63 95.25,75.56 v98.42,72.39 | v97.79,67.31 97.79,31.75 93.34,27.3 93.34,21.59 REFLET.2 97.16,17.78 97.16,6.99 91.44,1.27 85.09,1.27 83.82,2.54 83.82,14.61 82.55,15.88 81.92,15.24 80.01,15.24 79.38,15.88 78.11,15.88 77.47,15.24 v76.2,15.24 | ANALOG.7 43.18,59.69 39.37,59.69 38.1,60.96 36.83,59.69 36.83,58.42 38.1,57.15 v66.04,57.15 | v73.66,33.66 73.66,22.23 v76.2,19.68
  Bottom 0.305: v98.42,72.39 98.42,67.94 v97.79,67.31 | v66.04,57.15 67.31,57.15 71.12,53.34 71.12,36.2 v73.66,33.66 | v76.2,15.24 v76.2,19.68
A2  (via drill 0.48)
  Top 0.305: v38.73,87.63 38.73,92.08 43.81,97.16 62.23,97.16 v62.87,96.52 | v64.77,97.16 69.85,92.08 v76.2,92.08 | v86.36,92.08 90.17,92.08 IC4.9 | v74.93,54.61 74.93,58.42 67.94,65.41 66.67,65.41 64.77,67.31 64.77,74.3 62.87,76.2 62.87,88.9 62.23,89.53 62.23,92.08 v63.5,93.34
  Bottom 0.305: IC2.25 35.56,84.45 v38.73,87.63 | v64.77,97.16 64.14,96.52 v62.87,96.52 62.87,95.25 63.5,94.61 v63.5,93.34 | v86.36,92.08 v76.2,92.08 | JP5.3 74.93,49.53 v74.93,54.61
A02  (via drill 0.48)
  Top 0.305: IC4.15 77.47,92.08 81.28,88.27 81.28,85.72 85.72,81.28 v91.44,81.28 | v95.89,73.66 95.89,72.39 99.06,69.22 99.06,29.21 v97.16,27.3 | v71.12,55.88 v69.85,57.15 | v73.66,55.88 73.66,58.42 v72.39,59.69
  Bottom 0.305: v91.44,81.28 95.89,76.83 v95.89,73.66 | REFLET.3 97.16,24.13 v97.16,27.3 97.16,60.33 88.9,68.58 86.36,68.58 77.47,59.69 v72.39,59.69 | ANALOG.6 50.16,59.05 67.94,59.05 v69.85,57.15 | v73.66,55.88 v71.12,55.88
A3  (via drill 0.48)
  Top 0.305: v45.09,94.61 v40.01,89.53 | v78.11,64.77 78.11,55.88 78.74,55.24 78.74,52.07 | JP5.4 78.74,52.07 | DIST.1 88.9,24.77 88.9,29.84 78.74,40.01 78.74,52.07
  Bottom 0.305: IC2.26 33.02,83.19 39.37,89.53 v40.01,89.53 | v45.09,94.61 50.16,99.69 90.17,99.69 99.69,90.17 99.69,67.94 97.79,66.04 96.52,66.04 92.08,70.48 74.93,70.48 73.66,71.75 72.39,70.48 v78.11,64.77
A03  (via drill 0.48)
  Top 0.305: v96.52,86.36 96.52,76.83 99.69,73.66 99.69,28.57 95.89,24.77 REFLET.4 | v84.45,76.83 v84.45,68.58
  Bottom 0.305: 87.63,92.08 90.17,89.53 93.34,89.53 v96.52,86.36 | 87.63,92.08 IC4.12 | ANALOG.5 52.7,64.14 66.67,64.14 67.94,62.87 78.74,62.87 v84.45,68.58 | v84.45,76.83 84.45,78.74 83.82,79.38 83.82,88.27 87.63,92.08
A04  (via drill 0.48)
  Top 0.305: v86.36,67.31 v86.36,73.66 | v64.14,60.33 74.3,50.16 74.3,43.18 v87.63,29.84
  Bottom 0.305: IC4.1 74.93,85.09 v86.36,73.66 | v86.36,67.31 88.9,67.31 95.25,60.96 95.25,29.84 | REFLET.5 95.25,29.84 | ANALOG.4 54.61,59.69 63.5,59.69 v64.14,60.33 | 95.25,29.84 v87.63,29.84
A05  (via drill 0.48)
  Top 0.305: IC4.5 78.74,93.34 78.74,95.89 76.2,98.42 v68.58,98.42 | v27.3,95.89 22.86,91.44 22.86,85.72 17.78,80.64 v17.78,78.11 17.78,74.3 v14.61,71.12 | ANALOG.3 52.7,59.05 38.73,59.05 v38.1,59.69 | v31.11,65.41 26.04,65.41 24.13,63.5 v15.24,63.5
  Bottom 0.305: v68.58,98.42 67.94,98.42 67.31,99.06 50.8,99.06 45.09,93.34 32.38,93.34 29.84,95.89 v27.3,95.89 | v17.78,78.11 14.61,78.11 JP4.1 | v38.1,59.69 36.83,59.69 v31.11,65.41 | v15.24,63.5 14.61,64.14 v14.61,71.12
A06  (via drill 0.48)
  Top 0.305: v22.86,83.19 26.04,86.36 26.04,92.08 31.75,97.79 62.87,97.79 69.85,90.81 73.66,90.81 IC4.2 v73.03,82.55 | ANALOG.2 57.78,66.04 v57.15,66.67
  Bottom 0.305: v22.86,83.19 22.86,78.11 20.32,75.56 14.61,75.56 JP3.1 | v57.15,66.67 57.15,69.85 59.05,71.75 72.39,71.75 73.03,72.39 76.83,72.39 77.47,71.75 78.74,73.03 78.74,76.83 v73.03,82.55
A07  (via drill 0.48)
  Top 0.305: v78.74,83.19 74.93,83.19 v73.03,81.28 | v69.22,70.48 v69.22,73.66 | v59.69,70.48 59.69,62.23 ANALOG.1
  Bottom 0.305: v78.74,83.19 IC4.4 | v73.03,81.28 73.03,76.83 71.75,75.56 71.12,75.56 v69.22,73.66 | v69.22,70.48 61.59,70.48 60.96,71.12 60.33,71.12 v59.69,70.48
BUZZ  (via drill 0.48)
  Top 0.305: v15.24,92.71 JP1.1 | v28.57,93.34 36.83,85.09 48.9,85.09 BUZZER.+
  Bottom 0.305: v15.24,92.71 27.94,92.71 v28.57,93.34
CH  (via drill 0.48)
  Top 0.305: 19.68,85.72 19.68,87.63 20.95,88.9 S2.2 21.59,89.53 21.59,95.89 S2.1 | 19.68,85.72 v12.7,85.72 | 19.68,85.72 R4.1
  Bottom 0.305: v12.7,85.72 JP4.2
CTS
  Bottom 0.508: JP11.5 JP12.5
D2  (via drill 0.48)
  Top 0.305: IC2.4 35.56,66.04 v34.92,65.41 33.66,64.14 33.66,59.05 30.48,55.88 30.48,52.07 JP7.3 | v83.82,20.95 85.09,20.95 86.36,19.68 85.09,18.41 35.56,18.41 34.29,19.68 34.29,53.34 36.2,55.24 36.2,61.59 v37.47,62.87
  Bottom 0.305: ENC.3 83.82,15.88 v83.82,20.95 | v34.92,65.41 v37.47,62.87
D3  (via drill 0.48)
  Top 0.305: IC2.5 38.1,67.31 34.29,63.5 34.29,57.15 31.11,53.98 31.11,50.16 29.21,48.26 | v21.59,10.79 21.59,18.41 v24.77,21.59 | v24.77,34.92 24.77,41.27 25.4,41.91 25.4,48.9 23.5,50.8 24.77,52.07 28.57,48.26 29.21,48.26 | 29.21,48.26 JP7.4
  Bottom 0.305: ENC.4 92.71,15.88 97.16,11.43 97.16,6.99 92.71,2.54 70.48,2.54 58.42,14.61 31.75,14.61 27.94,10.79 v21.59,10.79 | v24.77,34.92 v24.77,21.59
D4  (via drill 0.48)
  Top 0.305: IC2.6 34.92,62.87 34.92,56.52 31.75,53.34 31.75,48.26 JP7.5 | v90.17,97.16 IC4.11 | v36.83,78.74 v30.48,85.09 | v30.48,72.39 v36.83,72.39 | v29.21,73.66 27.94,73.66 24.77,70.48 v24.13,70.48
  Bottom 0.305: v90.17,97.16 88.9,98.42 69.85,98.42 68.58,97.16 67.31,97.16 66.04,98.42 51.44,98.42 45.72,92.71 38.1,92.71 v30.48,85.09 | v36.83,72.39 v36.83,78.74 | v29.21,73.66 v30.48,72.39 | v24.13,70.48 24.13,67.31 24.77,66.67 24.77,64.14 24.13,63.5 24.13,52.7 26.67,50.16 26.67,46.99 JP7.5
D5  (via drill 0.48)
  Top 0.305: v50.16,71.75 50.16,73.03 52.07,74.93 52.07,78.74 53.34,80.01 52.07,81.28 40.64,81.28 36.83,77.47 30.48,83.82 JP9.1 | v25.4,72.39 23.5,74.3 23.5,82.55 v24.77,83.82
  Bottom 0.305: v50.16,71.75 IC2.11 | JP7.6 30.48,44.45 30.48,60.96 25.4,66.04 v25.4,72.39 | JP9.1 v24.77,83.82
D6  (via drill 0.48)
  Top 0.305: IC2.12 55.88,63.5 v56.52,62.87 | v62.23,61.59 59.05,58.42 v38.1,58.42 | JP9.2 24.77,82.55 v24.77,74.3
  Bottom 0.305: v56.52,62.87 57.15,62.87 57.78,63.5 60.33,63.5 v62.23,61.59 | 37.47,57.78 31.11,51.44 31.11,42.55 JP7.7 | 37.47,57.78 v38.1,58.42 | v24.77,74.3 29.21,69.85 29.21,66.04 37.47,57.78
D7  (via drill 0.48)
  Top 0.305: v68.58,66.67 73.66,66.67 74.3,66.04 79.38,66.04 87.63,57.78 87.63,55.88 NRF24L1.3 | JP7.8 31.75,40.64 31.75,46.99 33.66,48.9 33.66,53.98 35.56,55.88 35.56,62.23 39.37,66.04 40.64,66.04 41.27,66.67 41.91,66.67 42.55,66.04 50.8,66.04 52.07,67.31 52.07,69.85 53.34,71.12 55.88,71.12 IC2.13
  Bottom 0.305: IC2.13 60.96,66.04 67.94,66.04 v68.58,66.67
D8  (via drill 0.48)
  Top 0.305: IC2.14 66.04,63.5 v66.04,62.87 | JP8.1 29.84,33.66 31.75,31.75 31.75,18.41 34.29,15.88 74.3,15.88 76.2,17.78 85.72,17.78 90.17,22.23 90.17,42.55 87.63,45.09 v87.63,53.34
  Bottom 0.305: v66.04,62.87 70.48,58.42 82.55,58.42 83.19,59.05 84.45,59.05 NRF24L1.4 87.63,55.88 v87.63,53.34
D9  (via drill 0.48)
  Top 0.305: v53.98,83.19 IC2.15 | v47.62,83.19 34.29,83.19 JP9.3 | v33.02,15.88 v31.11,17.78 | v73.66,10.16 74.93,8.89 76.83,8.89 v82.55,14.61 | v88.9,22.23 88.9,23.5 89.53,24.13 89.53,41.91 81.92,49.53 v81.92,53.98 | v80.01,55.88 80.01,64.14 v79.38,64.77 | v67.94,76.2 v73.66,70.48
  Bottom 0.305: v47.62,83.19 v53.98,83.19 | JP8.2 31.11,28.57 v31.11,17.78 | v33.02,15.88 67.94,15.88 v73.66,10.16 | v82.55,14.61 82.55,20.95 83.82,22.23 85.72,20.32 87,20.32 v88.9,22.23 | v80.01,55.88 v81.92,53.98 | v73.66,70.48 v79.38,64.77 | v67.94,76.2 66.04,76.2 62.87,73.03 60.96,74.93 IC2.15
D10  (via drill 0.48)
  Top 0.305: IC2.16 50.16,84.45 35.56,84.45 JP9.4 | JP8.3 24.77,28.57 21.59,31.75 6.35,31.75 0.64,37.47 0.64,83.19 7.62,90.17 11.43,90.17 v12.7,91.44
  Bottom 0.305: JP9.4 v12.7,91.44
DTR
  Top 0.305: C3.2 19.05,56.52 JP11.1
  Bottom 0.508: JP11.1 JP12.1
GND  (via drill 0.48, 0.5)
  Top 0.762: IC3.2 69.85,12.06 D1.A C6.- 70.48,2.54 55.24,2.54 54.61,3.17 IC5.4 | U$13.P$3 U$13.P$1 | U$13.P$4 U$13.P$1 | U$13.P$5 U$13.P$1 | U$13.P$6 U$13.P$1 | U$13.P$7 U$13.P$1 | U$13.P$8 U$13.P$1 | U$13.P$9 U$13.P$1 | U$13.P$10 U$13.P$1 | U$13.P$11 U$13.P$1 | JP6.5 JP6.4 | U$15.P$2 U$15.P$1 | U$15.P$3 U$15.P$1 | U$15.P$4 U$15.P$1 | U$26.P$3 U$26.P$1 | U$26.P$4 U$26.P$1 | U$26.P$5 U$26.P$1 | U$26.P$6 U$26.P$1 | U$26.P$7 U$26.P$1 | U$26.P$8 U$26.P$1 | U$26.P$9 U$26.P$1 | U$26.P$10 U$26.P$1 | U$26.P$11 U$26.P$1 | v46.99,73.03 45.72,73.03 43.18,75.56 IC2.22 | IC4.6 IC4.7 IC4.8 | JP10.2 JP10.1 65.41,78.11 | C2.2 C1.2 65.41,75.56 65.41,78.11 | ICSP.6 85.72,77.47 85.09,78.11 65.41,78.11 | v59.69,83.82 53.34,90.17 50.8,90.17 48.26,87.63 BUZZER.- 40.64,87.63 39.37,86.36 37.47,86.36 v29.84,93.98 | 12.06,45.09 v13.97,45.09 IC1.2 | RESET.1 5.71,71.75 12.06,71.75 RESET.2 | S2.4 16.51,89.53 16.51,95.89 S2.3 | R7.A 31.11,4.45 27.94,1.27 12.06,1.27 10.16,3.17 10.16,10.79 12.06,12.7 ON.K | C5.- 22.23,34.29 14.61,34.29 C4.- 14.61,33.66 12.06,36.2 | 12.06,36.2 6.35,36.2 ALIM.1 | 12.06,36.2 12.06,45.09 | 12.06,45.09 IC1.4 | v70.48,23.5 U$26.P$1 | v71.12,14.61 32.38,14.61 JP8.7
  Bottom 0.762: JP12.6 5.08,57.15 | REFLET_ALIM.1 ENC.1 76.2,8.26 C6.- | NRF24L1.1 83.82,52.07 90.17,45.72 90.17,44.45 BUSS.1 77.47,31.75 | DIST.2 84.45,24.77 77.47,31.75 | U$26.P$12 U$15.P$5 | U$26.P$4 73.66,32.38 | 73.66,32.38 JP6.4 77.47,31.75 | U$15.P$1 U$13.P$12 | IC3.2 74.3,13.34 73.66,13.97 73.66,32.38 | IC2.8 45.72,71.75 v46.99,73.03 | BUZZER.- 43.81,76.83 IC2.22 | ICSP.6 89.53,86.36 IC4.7 | JP10.1 v59.69,83.82 | 15.24,15.24 15.88,15.88 26.04,15.88 JP8.7 | 15.24,15.24 12.7,12.7 ON.K | 12.7,31.75 12.7,27.94 RX.K 12.06,27.94 12.06,22.86 TX.K 12.7,22.86 13.97,21.59 13.97,16.51 15.24,15.24 | 12.7,31.75 14.61,33.66 C4.- | 12.7,31.75 12.7,48.9 JP11.6 5.08,57.15 | 5.08,57.15 3.81,57.15 3.17,57.78 3.17,67.31 5.08,69.22 5.08,71.12 RESET.1 5.08,71.75 5.08,74.93 3.17,76.83 3.17,90.81 R2.A 6.99,92.71 10.16,95.89 16.51,95.89 S2.3 17.14,95.89 19.05,93.98 27.3,93.98 27.94,94.61 29.21,94.61 v29.84,93.98 | v70.48,23.5 71.12,22.86 v71.12,14.61
  pour Bottom: 0,0 100.33,0 100.33,100.33 0,100.33
  pour Top: 0,0 100.33,0 100.33,100.33 0,100.33
GND1  (via drill 0.48)
  Top 0.762: v3.17,8.89 12.06,17.78 BAT.K
  Bottom 0.762: v3.17,8.89 10.79,1.27 38.73,1.27 47.62,10.16 IC5.7
LED_RX  (via drill 0.48)
  Top 0.305: R5.2 17.78,27.94 15.24,30.48 v4.45,30.48 | v4.45,65.41 v1.91,62.87
  Bottom 0.305: v4.45,30.48 4.45,53.34 1.27,56.52 1.27,62.23 v1.91,62.87 | v4.45,65.41 6.35,65.41 7.62,66.67 7.62,74.93 JP1.3
LED_TX  (via drill 0.48)
  Top 0.305: v16.51,38.73 v19.68,35.56 | v16.51,74.3 16.51,80.64 19.05,83.19 17.78,84.45 13.97,84.45 13.34,83.82 12.7,84.45 9.53,84.45 JP2.2
  Bottom 0.305: R3.2 23.5,26.04 19.68,29.84 v19.68,35.56 | v16.51,38.73 16.51,52.07 20.32,55.88 20.32,63.5 18.41,65.41 18.41,69.22 19.05,69.85 19.05,71.75 v16.51,74.3
MISO  (via drill 0.48)
  Top 0.305: IC2.18 55.88,73.66 60.96,73.66 62.23,74.93 62.23,88.27 61.59,88.9 61.59,92.71 v64.14,95.25 | 67.31,98.42 68.58,99.69 90.17,99.69 98.42,91.44 v98.42,87 | 67.31,98.42 v66.04,97.16 | NRF24L1.7 93.34,56.52 93.34,66.67 92.08,67.94 ICSP.1 | v26.67,34.92 26.67,48.9 v24.77,50.8 | v23.5,73.03 21.59,74.93 21.59,83.19 25.4,87 25.4,92.71 31.11,98.42 67.31,98.42
  Bottom 0.305: v66.04,97.16 v64.14,95.25 | v98.42,87 98.42,74.93 95.89,72.39 ICSP.1 | JP8.5 26.67,25.4 v26.67,34.92 | v24.77,50.8 22.86,52.7 22.86,72.39 v23.5,73.03
MOSI  (via drill 0.48)
  Top 0.305: v85.09,79.38 v71.75,79.38 | NRF24L1.6 88.9,63.5 87.63,64.77 87.63,73.03 ICSP.4 | JP8.4 24.77,26.04 20.32,21.59 v20.32,10.79 | v33.66,13.34 73.03,13.34 76.2,16.51 83.19,16.51 84.45,15.24 84.45,6.99 85.09,6.35 87.63,6.35 91.44,10.16 v91.44,43.81
  Bottom 0.305: IC2.17 59.05,79.38 v71.75,79.38 | ICSP.4 v85.09,79.38 | v20.32,10.79 21.59,9.53 29.84,9.53 v33.66,13.34 | v91.44,43.81 91.44,52.7 90.17,53.98 90.17,55.88 NRF24L1.6
N$1
  Top 0.305: R3.1 13.97,20.95 12.06,20.95 10.16,22.86 TX.A
N$2
  Top 0.305: R5.1 13.97,29.84 12.06,29.84 10.16,27.94 RX.A
N$3  (via drill 0.9 pad 1.68)
  other vias: 64.14,29.84
N$4  (via drill 0.9 pad 1.68)
  other vias: 66.67,29.84
N$5  (via drill 0.9 pad 1.68)
  other vias: 41.27,52.7
N$6
  Top 0.305: C2.1 77.47,68.58 Q1.1
  Bottom 0.305: IC2.10 53.98,65.41 68.58,65.41 C2.1
N$7  (via drill 0.9 pad 1.68)
  other vias: 48.9,19.68
N$8
  Bottom 1.016: ALIM.2 6.35,13.34 11.43,8.26 12.7,8.26 15.24,5.71 S1.2
N$9  (via drill 0.5)
  other vias: 6.99,48.26
N$10  (via drill 0.9 pad 1.68)
  other vias: 46.35,19.68
N$11
  Bottom 0.305: IC2.9 48.26,71.12 51.44,74.3 52.7,74.3 54.61,72.39 69.85,72.39 71.12,73.66 | C1.1 71.12,73.66 | 71.12,73.66 77.47,73.66 Q1.2
N$12  (via drill 0.5)
  other vias: 6.99,45.09
N$13  (via drill 0.9 pad 1.68)
  other vias: 41.27,29.84
N$14  (via drill 0.9 pad 1.68)
  other vias: 38.73,29.84
N$15  (via drill 0.5)
  other vias: 6.99,41.91
N$16  (via drill 0.5)
  other vias: 13.97,41.91
N$17  (via drill 0.5)
  other vias: 13.97,48.26
N$18  (via drill 0.9 pad 1.68)
  other vias: 64.14,27.3
N$19  (via drill 0.9 pad 1.68)
  other vias: 66.67,27.3
N$23  (via drill 0.9 pad 1.68)
  other vias: 64.14,34.92
N$25  (via drill 0.9 pad 1.68)
  other vias: 48.9,17.14
N$26  (via drill 0.9 pad 1.68)
  other vias: 46.35,17.14
N$27  (via drill 0.9 pad 1.68)
  other vias: 43.81,17.14
N$30  (via drill 0.9 pad 1.68)
  other vias: 66.67,34.92
N$31  (via drill 0.9 pad 1.68)
  other vias: 64.14,32.38
N$32  (via drill 0.9 pad 1.68)
  other vias: 41.27,27.3
N$33  (via drill 0.9 pad 1.68)
  other vias: 38.73,27.3
N$34  (via drill 0.9 pad 1.68)
  other vias: 66.67,32.38
N$35  (via drill 0.9 pad 1.68)
  other vias: 43.73,19.7
N$47  (via drill 0.9 pad 1.68)
  other vias: 64.14,40.01
N$49  (via drill 0.9 pad 1.68)
  other vias: 66.67,40.01
N$52  (via drill 0.9 pad 1.68)
  other vias: 64.14,37.47
N$53  (via drill 0.9 pad 1.68)
  other vias: 66.67,37.47
N$55
  Top 0.762: U$3.P$2 U$3.P$1
N$56
  Top 0.762: U$4.P$2 U$4.P$1
N$57
  Top 0.762: U$5.P$2 U$5.P$1
N$58
  Top 0.762: U$6.P$2 U$6.P$1
N$59
  Top 0.762: U$7.P$2 U$7.P$1
N$62  (via drill 0.9 pad 1.68)
  other vias: 36.2,19.68
N$63  (via drill 0.9 pad 1.68)
  other vias: 36.2,17.14
N$65  (via drill 0.9 pad 1.68)
  other vias: 41.27,34.92
N$66  (via drill 0.9 pad 1.68)
  other vias: 38.73,34.92
N$67  (via drill 0.9 pad 1.68)
  other vias: 36.2,22.23
N$68  (via drill 0.9 pad 1.68)
  other vias: 41.27,32.38
N$69  (via drill 0.9 pad 1.68)
  other vias: 38.73,32.38
N$70
  Top 0.762: U$8.P$2 U$8.P$1
N$78  (via drill 0.9 pad 1.68)
  other vias: 41.27,40.01
N$79  (via drill 0.9 pad 1.68)
  other vias: 38.73,40.01
N$80
  Top 0.762: U$9.P$2 U$9.P$1
N$82  (via drill 0.9 pad 1.68)
  other vias: 64.14,45.09
N$83  (via drill 0.9 pad 1.68)
  other vias: 66.67,45.09
N$84  (via drill 0.9 pad 1.68)
  other vias: 64.14,42.55
N$87  (via drill 0.9 pad 1.68)
  other vias: 66.67,42.55
N$88
  Top 0.762: U$10.P$2 U$10.P$1
N$89
  Top 0.762: U$11.P$2 U$11.P$1
N$92
  Top 0.762: U$17.P$2 U$17.P$1
N$93
  Top 0.762: U$18.P$2 U$18.P$1
N$94
  Top 0.762: U$19.P$2 U$19.P$1
N$95  (via drill 0.9 pad 1.68)
  other vias: 56.52,47.62
N$96  (via drill 0.9 pad 1.68)
  other vias: 59.05,47.62
N$97  (via drill 0.9 pad 1.68)
  other vias: 41.27,37.47
N$98  (via drill 0.9 pad 1.68)
  other vias: 38.73,37.47
N$99  (via drill 0.9 pad 1.68)
  other vias: 61.59,47.62
N$101  (via drill 0.9 pad 1.68)
  other vias: 64.14,50.16
N$102  (via drill 0.9 pad 1.68)
  other vias: 66.67,50.16
N$103  (via drill 0.9 pad 1.68)
  other vias: 64.14,47.62
N$104  (via drill 0.9 pad 1.68)
  other vias: 66.67,47.62
N$111  (via drill 0.9 pad 1.68)
  other vias: 56.52,50.16
N$112  (via drill 0.9 pad 1.68)
  other vias: 59.05,50.16
N$113  (via drill 0.9 pad 1.68)
  other vias: 61.59,50.16
N$115
  Top 0.762: U$20.P$2 U$20.P$1
N$116
  Top 0.762: U$21.P$2 U$21.P$1
N$117
  Top 0.762: U$22.P$2 U$22.P$1
N$120
  Top 0.762: U$23.P$2 U$23.P$1
N$121
  Top 0.762: U$24.P$2 U$24.P$1
N$122
  Top 0.762: U$25.P$2 U$25.P$1
N$124
  Top 0.762: U$2.P$2 U$2.P$1
N$125  (via drill 0.9 pad 1.68)
  other vias: 56.52,52.7
N$126
  Top 0.762: U$16.P$2 U$16.P$1
N$127  (via drill 0.9 pad 1.68)
  other vias: 66.67,52.7
N$128  (via drill 0.9 pad 1.68)
  other vias: 43.81,52.7
N$129  (via drill 0.9 pad 1.68)
  other vias: 64.14,19.68
N$130  (via drill 0.9 pad 1.68)
  other vias: 41.27,45.09
N$131  (via drill 0.9 pad 1.68)
  other vias: 38.73,45.09
N$132  (via drill 0.9 pad 1.68)
  other vias: 46.35,52.7
N$133  (via drill 0.9 pad 1.68)
  other vias: 41.27,42.55
N$134  (via drill 0.9 pad 1.68)
  other vias: 38.73,42.55
N$135  (via drill 0.9 pad 1.68)
  other vias: 66.67,19.68
N$136  (via drill 0.9 pad 1.68)
  other vias: 64.14,17.14
N$137  (via drill 0.9 pad 1.68)
  other vias: 66.67,17.14
N$138  (via drill 0.9 pad 1.68)
  other vias: 48.9,47.62
N$139  (via drill 0.9 pad 1.68)
  other vias: 46.35,47.62
N$140  (via drill 0.9 pad 1.68)
  other vias: 43.81,47.62
N$141  (via drill 0.9 pad 1.68)
  other vias: 64.14,24.77
N$142  (via drill 0.9 pad 1.68)
  other vias: 66.67,24.77
N$143  (via drill 0.9 pad 1.68)
  other vias: 41.27,50.16
N$144  (via drill 0.9 pad 1.68)
  other vias: 38.73,50.16
N$145  (via drill 0.9 pad 1.68)
  other vias: 64.14,22.23
N$146  (via drill 0.9 pad 1.68)
  other vias: 66.67,22.23
N$147  (via drill 0.9 pad 1.68)
  other vias: 64.14,52.7
N$148  (via drill 0.9 pad 1.68)
  other vias: 61.59,52.7
N$149  (via drill 0.9 pad 1.68)
  other vias: 59.05,52.7
N$150  (via drill 0.9 pad 1.68)
  other vias: 53.98,19.68
N$151  (via drill 0.9 pad 1.68)
  other vias: 53.98,17.14
N$155  (via drill 0.9 pad 1.68)
  other vias: 56.52,17.14
N$156  (via drill 0.9 pad 1.68)
  other vias: 59.05,17.14
N$157  (via drill 0.9 pad 1.68)
  other vias: 61.59,17.14
N$158  (via drill 0.9 pad 1.68)
  other vias: 56.52,19.68
N$159  (via drill 0.9 pad 1.68)
  other vias: 59.05,19.68
N$160  (via drill 0.9 pad 1.68)
  other vias: 61.68,19.7
N$162  (via drill 0.9 pad 1.68)
  other vias: 41.27,47.62
N$163  (via drill 0.9 pad 1.68)
  other vias: 38.73,47.62
N$164  (via drill 0.9 pad 1.68)
  other vias: 69.22,19.68
N$165  (via drill 0.9 pad 1.68)
  other vias: 69.22,17.14
N$166  (via drill 0.9 pad 1.68)
  other vias: 69.22,22.23
N$172  (via drill 0.9 pad 1.68)
  other vias: 51.44,19.68
N$173  (via drill 0.9 pad 1.68)
  other vias: 48.9,50.16
N$174  (via drill 0.9 pad 1.68)
  other vias: 46.35,50.16
N$175  (via drill 0.9 pad 1.68)
  other vias: 43.81,50.16
N$185
  Top 0.305: R9.1 13.97,19.68 12.06,19.68 10.16,17.78 BAT.A
N$186
  Top 0.305: R1.1 13.97,14.61 12.06,14.61 10.16,12.7 ON.A
N$189
  Top 0.762: R8.1 62.23,4.45 D1.C
  Bottom 0.762: IC5.6 50.16,10.16 52.07,8.26 55.88,8.26 D1.C
N$190
  Bottom 0.762: R7.S 44.45,13.34 50.8,13.34 52.7,11.43 IC5.5
N$195  (via drill 0.9 pad 1.68)
  other vias: 51.44,17.14
N$198  (via drill 0.9 pad 1.68)
  other vias: 48.9,52.7
N$199  (via drill 0.9 pad 1.68)
  other vias: 38.73,52.7
N$208  (via drill 0.9 pad 1.68)
  other vias: 41.27,19.68
N$209  (via drill 0.9 pad 1.68)
  other vias: 38.73,19.68
N$227  (via drill 0.9 pad 1.68)
  other vias: 41.27,17.14
N$228  (via drill 0.9 pad 1.68)
  other vias: 38.73,17.14
N$260  (via drill 0.9 pad 1.68)
  other vias: 41.27,24.77
N$261  (via drill 0.9 pad 1.68)
  other vias: 38.73,24.77
N$263  (via drill 0.9 pad 1.68)
  other vias: 41.27,22.23
N$264  (via drill 0.9 pad 1.68)
  other vias: 38.73,22.23
POT
  Bottom 0.305: R2.S 7.62,85.09 JP3.2
RES  (via drill 0.48)
  Top 0.305: v1.91,64.14 5.08,67.31 RESET.3 5.71,67.31 12.06,67.31 RESET.4 12.7,66.67 13.34,66.04 R6.1 22.23,68.58 IC2.1 | JP6.1 81.92,19.68 v85.09,19.68 | v93.34,67.94 93.34,71.75 93.98,72.39 93.98,75.56 ICSP.5 | v27.3,2.54 31.11,6.35 35.56,6.35 39.37,2.54 42.55,2.54 44.45,0.64 92.08,0.64 v97.79,6.35
  Bottom 0.305: IC2.1 27.94,65.41 C3.1 | v1.91,64.14 0.64,62.87 0.64,55.88 1.91,54.61 1.91,12.06 11.43,2.54 v27.3,2.54 | v85.09,19.68 90.17,19.68 94.61,15.24 95.89,15.24 97.79,17.14 | 97.79,17.14 98.42,17.78 98.42,62.87 v93.34,67.94 | 97.79,17.14 v97.79,6.35
RX  (via drill 0.48)
  Top 0.305: IC2.2 30.48,67.31 32.38,65.41 32.38,62.23 v28.57,58.42 22.23,58.42 18.41,54.61 v17.78,54.61 | JP1.2 3.17,78.11 3.17,71.75 6.35,68.58 15.88,68.58 v17.14,67.31
  Bottom 0.305: JP7.1 v28.57,58.42 | v17.14,67.31 17.14,65.41 19.68,62.87 19.68,56.52 v17.78,54.61 14.61,54.61 JP11.3
  Bottom 0.508: JP11.3 JP12.3
SCK  (via drill 0.48)
  Top 0.305: v71.75,80.64 72.39,80.64 73.03,80.01 84.45,80.01 85.09,80.64 90.81,80.64 93.98,77.47 | 93.98,77.47 94.61,76.83 94.61,55.88 92.08,53.34 90.17,53.34 NRF24L1.5 | JP8.6 30.48,22.86 v30.48,31.75 | v33.02,42.55 v33.02,34.29 | v31.75,71.12 36.83,71.12 v39.37,73.66 | v42.55,78.74 48.9,78.74 50.8,76.83 IC2.19 | 93.98,77.47 v93.98,76.83
  Bottom 0.305: IC2.19 55.24,80.64 v71.75,80.64 | v33.02,34.29 v30.48,31.75 | v33.02,42.55 33.02,52.07 39.37,58.42 39.37,59.69 31.75,67.31 v31.75,71.12 | v39.37,73.66 39.37,77.47 40.64,78.74 v42.55,78.74 | v93.98,76.83 ICSP.3
SCL  (via drill 0.48)
  Top 0.305: v40.64,64.14 52.7,64.14 54.61,66.04 v54.61,66.67 | v52.7,73.03 61.59,73.03 v62.87,74.3 | v71.12,76.83 78.74,69.22 78.74,67.94 78.11,67.31 v74.3,67.31 | v74.3,64.14 74.3,60.33 76.83,57.78 JP5.6
  Bottom 0.305: IC2.28 34.29,69.85 34.29,67.31 37.47,64.14 v40.64,64.14 | v54.61,66.67 54.61,71.12 v52.7,73.03 | v62.87,74.3 66.04,77.47 70.48,77.47 v71.12,76.83 | v74.3,64.14 v74.3,67.31 | BUSS.4 83.82,48.26 JP5.6
SDA  (via drill 0.48)
  Top 0.305: v52.7,65.41 v41.91,65.41 | v67.94,64.14 67.94,60.33 75.56,52.7 JP5.5
  Bottom 0.305: IC2.27 36.83,69.85 36.83,67.31 38.73,65.41 v41.91,65.41 | v52.7,65.41 53.34,64.77 67.31,64.77 v67.94,64.14 | BUSS.3 78.74,48.26 78.74,50.8 JP5.5
TX  (via drill 0.48)
  Top 0.305: JP2.1 9.53,78.11 12.7,78.11 v17.78,83.19 | v26.04,75.56 v26.04,81.28 | v30.48,71.12 IC2.3 33.02,61.59 26.67,55.24 26.67,54.61 27.94,53.34 | JP11.2 16.51,55.24 16.51,54.61 17.78,53.34 27.94,53.34 | 27.94,53.34 JP7.2
  Bottom 0.305: v17.78,83.19 21.59,83.19 22.86,84.45 v26.04,81.28 | v30.48,71.12 v26.04,75.56
  Bottom 0.508: JP11.2 JP12.2

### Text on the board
tPlace: ROBO F v3 | REV 1 | 0 | 1 | 2 | 3 | 4 | 5 | 6 | 7 | GND | CTS | 5V | RX | TX | DTR | LOW
tNames: EXTRA | 5V | GND | 5V | GND | NRF24L01 | GND | 5V
tDocu: Fernando Padilha Ferreira

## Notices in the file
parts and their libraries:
SparkFun-Connectors: Licensing: CC v3.0 Share-Alike You are welcome to use this library for commercial purposes.
SparkFun-Aesthetics: Released under the Creative Commons Attribution Share-Alike 3.0 License
SparkFun-Aesthetics: http://creativecommons.org/licenses/by-sa/3.0
